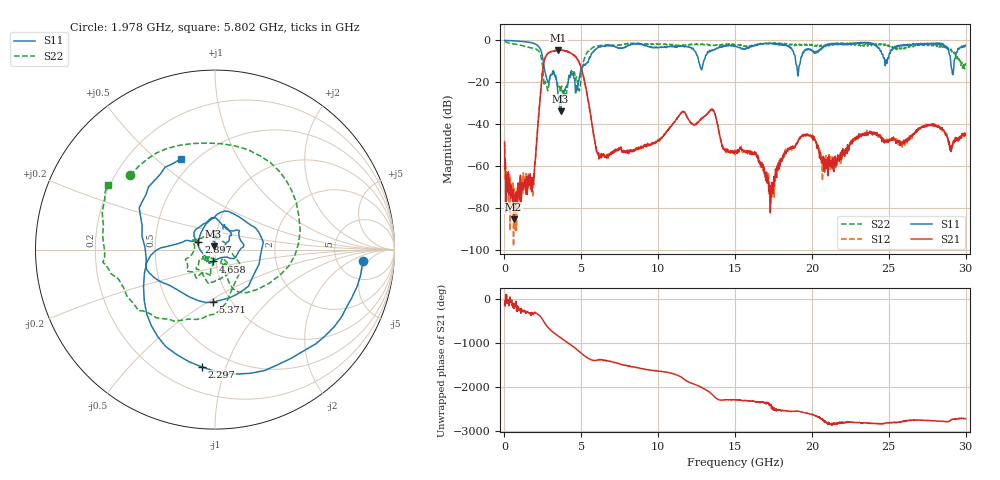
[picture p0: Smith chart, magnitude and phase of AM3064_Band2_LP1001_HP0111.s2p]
# Hz S DB R 50.0
!freq dBS11 angS11 dBS21 angS21 dBS12 angS12 dBS22 angS22
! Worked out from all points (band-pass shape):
!   1600 points, 10 MHz to 29.98 GHz, reference 50 ohm
!   highest |S21| = -4.57 dB at 3.515 GHz (marker M1); lowest = -85.3 dB at 591.1 MHz (marker M2)
!   |S21| within 3 dB of the highest: 2.689 GHz to 4.589 GHz (1.899 GHz wide, 52.2 % of centre)
!   lowest |S11| = -33.8 dB at 3.646 GHz (marker M3), VSWR 1.04, Z = 49.2 + j1.83 ohm
!   |S11| at or under -10 dB: 2.531 GHz to 5.459 GHz (2.928 GHz wide, 73.3 % of centre); 12.63 GHz to 12.96 GHz (324.5 MHz wide, 2.54 % of centre); 18.94 GHz to 19.25 GHz (305.1 MHz wide, 1.6 % of centre)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
!   |S22| runs from -26.8 to -0.3 dB; largest |S21 - S12| = 0.017
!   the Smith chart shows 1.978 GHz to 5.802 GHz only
!   S11 on the Smith chart (normalised r, x): 1.978 GHz: 9.11, -3.49; 2.297 GHz: 0.36, -0.83; 2.897 GHz: 0.83, +0.07; 4.658 GHz: 0.97, -0.13; 5.371 GHz: 0.82, -0.53; 5.802 GHz: 0.42, +0.61
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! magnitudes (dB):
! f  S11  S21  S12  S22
! 10 MHz  0.0  -49.0  -47.8  -0.3
! 591.1 MHz  -0.2  -85.3  -98.1  -1.7
! 1.978 GHz  -1.7  -58.1  -59.0  -4.0
! 2.297 GHz  -3.6  -29.1  -29.2  -6.0
! 2.897 GHz  -19.8  -5.8  -5.8  -20.5
! 3.515 GHz  -27.1  -4.6  -4.7  -22.5
! 3.646 GHz  -33.8  -4.7  -4.7  -24.6
! 4.658 GHz  -23.4  -8.2  -7.9  -18.0
! 5.015 GHz  -12.9  -13.7  -13.7  -14.8
! 5.371 GHz  -10.7  -25.7  -25.5  -5.9
! 5.802 GHz  -5.3  -44.9  -45.3  -3.2
! 6.627 GHz  -2.5  -55.9  -56.1  -2.3
! 10 GHz  -3.4  -47.6  -47.4  -1.8
! 13.49 GHz  -4.6  -33.1  -32.8  -2.2
! 15 GHz  -2.5  -53.4  -53.8  -1.9
! 16.32 GHz  -2.3  -54.0  -54.0  -2.1
! 17.4 GHz  -1.7  -67.7  -69.6  -1.3
! 18.29 GHz  -2.3  -53.4  -51.9  -1.9
! 19.99 GHz  -4.5  -45.9  -46.1  -1.9
! 20.82 GHz  -2.8  -56.4  -59.5  -2.4
! 25 GHz  -7.9  -48.5  -47.7  -2.2
! 29.98 GHz  -2.3  -44.8  -45.0  -10.8
